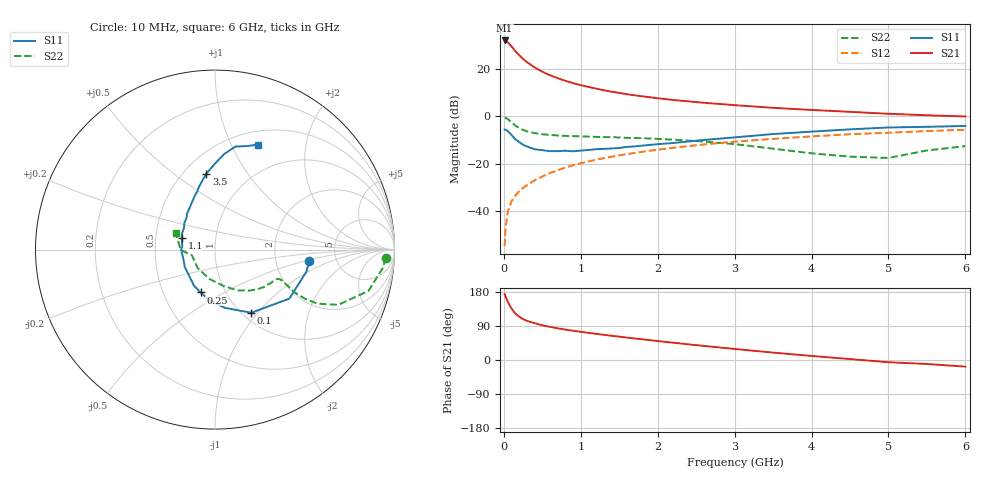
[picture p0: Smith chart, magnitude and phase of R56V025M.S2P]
! SIEMENS Small Signal Semiconductors
! BFR183
! Si NPN RF Bipolar Junction Transistor in SOT23
! VCE = 6 V  IC = 25 mA
! Common Emitter S-Parameters:  May  1996
# GHz  S  MA  R  50
!  f  S11  S21  S12  S22
! GHz  MAG  ANG  MAG  ANG  MAG  ANG  MAG  ANG
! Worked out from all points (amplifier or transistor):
!   36 points, 10 MHz to 6 GHz, reference 50 ohm
!   highest |S21| = 32.2 dB at 10 MHz (marker M1)
!   |S21| within 3 dB of that: start of sweep to 112 MHz
!   unconditionally stable (mu >= 1): 534.7 MHz to 2.431 GHz
!   at 250 MHz: K = 0.84, MSG = 27.3 dB, |S12| = -30.2 dB
!   at 1.4 GHz: K = 1.04, MAG = 12.5 dB, |S12| = -17.0 dB
!   at 6 GHz: K = 0.90, MSG = 2.8 dB, |S12| = -5.6 dB
!   S11 on the Smith chart (normalised r, x): 10 MHz: 3.14, -0.55; 100 MHz: 1.10, -0.93; 250 MHz: 0.76, -0.39; 1.1 GHz: 0.68, +0.09; 3.5 GHz: 0.64, +0.66; 6 GHz: 0.65, +1.27
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0.01  0.5288 -6.9  40.67 174.1  0.0018 93.8  0.9536 -2.8
0.02  0.5243 -13.5  40.15 168.6  0.0038 84.4  0.9394 -6.4
0.05  0.4963 -33.4  37.28 154.3  0.0095 76.5  0.8858 -15.0
0.1  0.4058 -60.1  30.4 135.6  0.0161 71.0  0.7536 -24.1
0.15  0.3294 -80.3  24.24 122.6  0.0212 69.1  0.6433 -27.9
0.2  0.2877 -95.3  19.84 114.2  0.0263 69.6  0.5699 -28.6
0.25  0.2517 -108.7  16.54 108.0  0.0308 69.7  0.5181 -28.4
0.3  0.2323 -120.5  14.15 103.4  0.0351 70.8  0.4852 -27.7
0.4  0.2025 -136.6  10.95 97.1  0.0446 71.6  0.4448 -26.2
0.5  0.1939 -150.6  8.858 91.6  0.0539 72.5  0.4202 -25.1
0.6  0.1844 -161.4  7.48 87.4  0.0634 72.5  0.4067 -24.6
0.7  0.1844 -171.2  6.476 83.6  0.073 72.8  0.3967 -24.6
0.8  0.1884 180.0  5.677 80.2  0.0827 71.9  0.3891 -24.9
0.9  0.1832 173.3  5.075 77.2  0.0927 71.3  0.3833 -25.2
1.1  0.1954 161.2  4.219 71.7  0.1117 69.9  0.375 -27.2
1.3  0.2063 150.8  3.593 66.5  0.1314 68.2  0.3669 -29.1
1.6  0.2267 138.6  2.962 59.0  0.1599 65.2  0.3534 -33.2
2.2  0.2746 120.5  2.237 45.7  0.2175 58.8  0.3243 -43.1
3.5  0.4253 96.6  1.525 19.5  0.3358 42.3  0.2082 -76.8
4.5  0.5343 84.6  1.254 2.5  0.4211 29.8  0.1414 -132.2
5.5  0.6042 72.7  1.062 -10.5  0.4915 18.3  0.1912 -179.3
6  0.6315 67.8  0.999 -17.5  0.5248 10.9  0.2361 157.4
